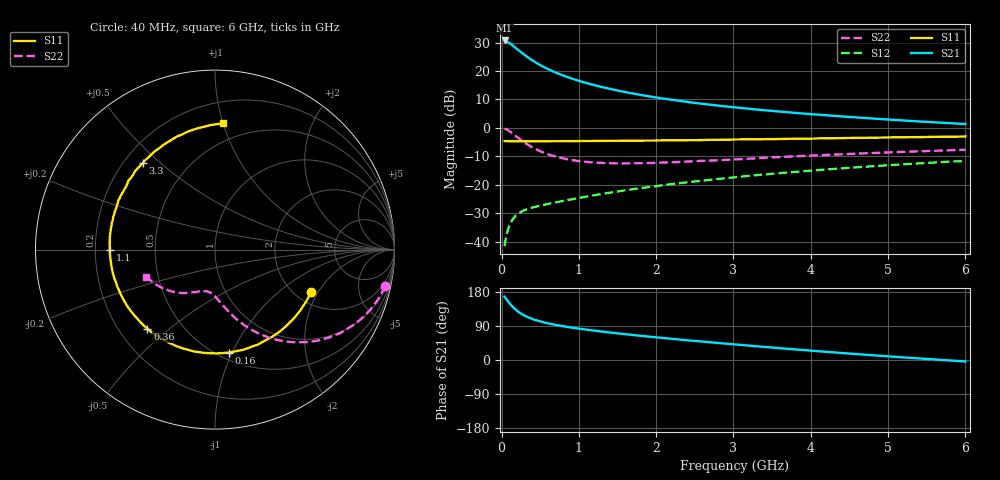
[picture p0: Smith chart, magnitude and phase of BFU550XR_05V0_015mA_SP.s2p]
! Filename:  P:\Prog\Test\Noise\ATS_data\Testdata_Net\03 Spar\BFU550XR_APG2013_45_C05_05p0V_015mA_SP_CM01_D.s2p
! Date/Time: Tue 06/Aug/2013 14:38:16
! BFU550XR_APG2013_45_C05_05p0V_1to35mA_SP_CM01_Bias6_R.s2p
! MDIF S-parameter v. bias file
! BFU550XR_APG2013_45_C05_05p0V_1to35mA_SP_CM01
! Date/time Fri Aug 02 14:46:46 2013
! VAR V_out= 5.0000
! VAR I_out= 14.9950
! VAR V_in= 0.8286
! VAR I_in= 0.1663
! Device data file deembeded for feedlines and parallel
! Original file: \03 Spar\BFU550XR_APG2013_45_C05_05p0V_015mA_SP_CM01_R.s2p
! Feed-files: PR006V01_02082013_Feed1.s2p, PR006V01_02082013_Feed2.s2p
! Parallel-file: PR006V01_02082013_Par.s2p
# MHz S MA R 50
!  Freq-MHz  S11-mag  S11-arg  S21-mag  S21-arg  S12-mag  S12-arg  S22-mag  S22-arg
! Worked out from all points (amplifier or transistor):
!   98 points, 40 MHz to 6 GHz, reference 50 ohm
!   highest |S21| = 30.7 dB at 40 MHz (marker M1)
!   |S21| within 3 dB of that: start of sweep to 199.9 MHz
!   unconditionally stable (mu >= 1): 1.646 GHz to 3.63 GHz
!   at 300 MHz: K = 0.37, MSG = 27.3 dB, |S12| = -28.9 dB
!   at 1.6 GHz: K = 0.99, MSG = 17.3 dB, |S12| = -22.0 dB
!   at 6 GHz: K = 0.88, MSG = 6.5 dB, |S12| = -11.6 dB
!   S11 on the Smith chart (normalised r, x): 40 MHz: 2.42, -1.75; 160 MHz: 0.56, -0.98; 360 MHz: 0.32, -0.42; 1.1 GHz: 0.26, -0.00; 3.3 GHz: 0.28, +0.44; 6 GHz: 0.36, +1.00
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40  0.5862 -23.8  34.43 167.2  0.008292 80.4  0.9672 -12.1
50  0.5844 -29.6  34.12 163.7  0.01028 77.9  0.9584 -15.1
80  0.5822 -46.1  32.34 155.7  0.01562 71.4  0.9128 -23.6
100  0.5812 -56.3  31.09 150.5  0.01876 67.6  0.8768 -28.7
120  0.5804 -65.8  29.81 145.6  0.02158 64.0  0.84 -33.5
160  0.5792 -82.1  26.98 137.2  0.02625 58.4  0.7634 -41.7
200  0.5787 -95.8  24.37 130.1  0.02977 54.1  0.6907 -48.4
260  0.5793 -111.8  20.99 121.6  0.03368 49.9  0.5996 -56.4
300  0.5796 -120.4  19.08 117.0  0.03572 48.0  0.5491 -60.6
360  0.5802 -130.5  16.66 111.5  0.03821 46.2  0.4873 -65.8
460  0.5803 -143.1  13.65 104.3  0.04166 45.1  0.4117 -72.2
600  0.5811 -155.5  10.83 96.8  0.04586 45.4  0.3429 -78.6
800  0.5842 -167.4  8.308 89.0  0.052 47.0  0.2898 -85.2
1050  0.5864 -178.0  6.412 81.4  0.06007 49.5  0.2557 -91.1
1100  0.5862 -179.9  6.129 80.1  0.06176 49.8  0.2518 -92.2
1500  0.5916 168.0  4.538 70.3  0.07596 52.0  0.2375 -99.5
2050  0.6 154.9  3.336 58.9  0.0964 52.7  0.2439 -107.8
3100  0.6257 133.5  2.236 39.7  0.1389 50.2  0.2818 -121.7
3300  0.6278 129.8  2.102 36.1  0.1472 49.1  0.292 -124.0
4100  0.651 116.0  1.703 23.1  0.181 44.5  0.329 -134.4
5200  0.683 98.2  1.348 6.8  0.2288 36.4  0.3782 -148.3
6000  0.7048 86.3  1.167 -3.8  0.2621 29.8  0.4111 -158.6
